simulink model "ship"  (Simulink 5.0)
settings: Solver=ode45  StartTime=0.0  StopTime=10.0  RelTol=1e-3
libraries: simulink x2

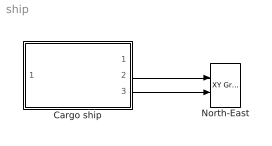
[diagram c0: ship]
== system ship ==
  Cargo ship : Subsystem  mask(Simple shipmodel for a cargo ship){current=off, noise=on, logic=on}
      mask prompts: current "current (in deg)"; noise "measurement noise"; logic "waves"
      mask help: Measurement noise: checked = noise on unchecked = noise off Current: checked = current on unchecked = current off Waves: checked = waves on unchecked = waves off Author: Jørgen Spjøtvold, 9/10-2003 TTK 4115 Linear system theory.
  North-East : simulink/Sinks/XY Graph  xmin=-5000  xmax=5000  ymin=-5000  ymax=5000  st=-1
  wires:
  Cargo ship/3(x) -> North-East/2
  Cargo ship/2(y) -> North-East/1

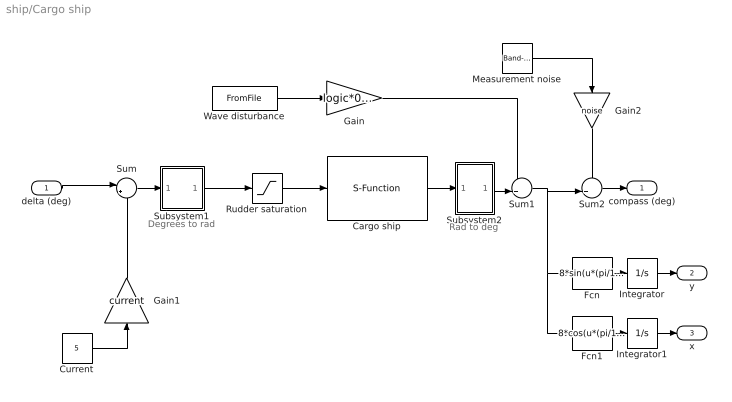
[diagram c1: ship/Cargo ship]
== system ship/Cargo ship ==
  note: Degrees to rad
  note: Rad to deg
  delta (deg) : Inport
  Cargo ship : S-Function  FunctionName=Shipmodel
  Current : Constant  Value=5
  Fcn : Fcn  Expr=8*sin(u*(pi/180))
  Fcn1 : Fcn  Expr=8*cos(u*(pi/180))
  Gain : Gain  Gain=logic*0.5
  Gain1 : Gain  Orientation=up  Gain=current
  Gain2 : Gain  Orientation=down  Gain=noise
  Integrator : Integrator
  Integrator1 : Integrator
  Measurement noise : simulink/Sources/Band-Limited White Noise  Cov=[0.001]  Ts=0.5  seed=[23341]
  Rudder saturation : Saturate  UpperLimit=45*(pi/180)  LowerLimit=-45*(pi/180)
  Subsystem1 : Subsystem
  Subsystem2 : Subsystem
  Sum : Sum  Inputs=|+-
  Sum1 : Sum  Inputs=++|
  Sum2 : Sum  Inputs=++|
  Wave disturbance : FromFile  FileName=wave.mat  SampleTime=0
  compass (deg) : Outport
  y : Outport  Port=2
  x : Outport  Port=3
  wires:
  Sum/1 -> Subsystem1/1(In1)
  delta (deg)/1 -> Sum/1
  Fcn/1 -> Integrator/1
  Integrator/1 -> y/1
  Fcn1/1 -> Integrator1/1
  Integrator1/1 -> x/1
  Wave disturbance/1 -> Gain/1
  Subsystem2/1(Out1) -> Sum1/2
  Gain/1 -> Sum1/1
  Sum1/1 -> Fcn/1, Fcn1/1, Sum2/2
  Current/1 -> Gain1/1
  Cargo ship/1 -> Subsystem2/1(In1)
  Subsystem1/1(Out1) -> Rudder saturation/1
  Gain1/1 -> Sum/2
  Rudder saturation/1 -> Cargo ship/1
  Sum2/1 -> compass (deg)/1
  Measurement noise/1 -> Gain2/1
  Gain2/1 -> Sum2/1

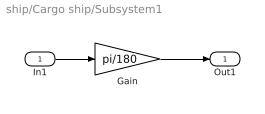
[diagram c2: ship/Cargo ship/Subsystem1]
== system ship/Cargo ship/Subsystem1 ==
  In1 : Inport
  Gain : Gain  Gain=pi/180
  Out1 : Outport
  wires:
  Gain/1 -> Out1/1
  In1/1 -> Gain/1

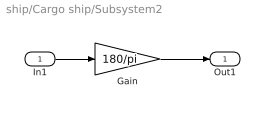
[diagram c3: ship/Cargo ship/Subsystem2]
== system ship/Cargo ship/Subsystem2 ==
  In1 : Inport
  Gain : Gain  Gain=180/pi
  Out1 : Outport
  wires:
  Gain/1 -> Out1/1
  In1/1 -> Gain/1
